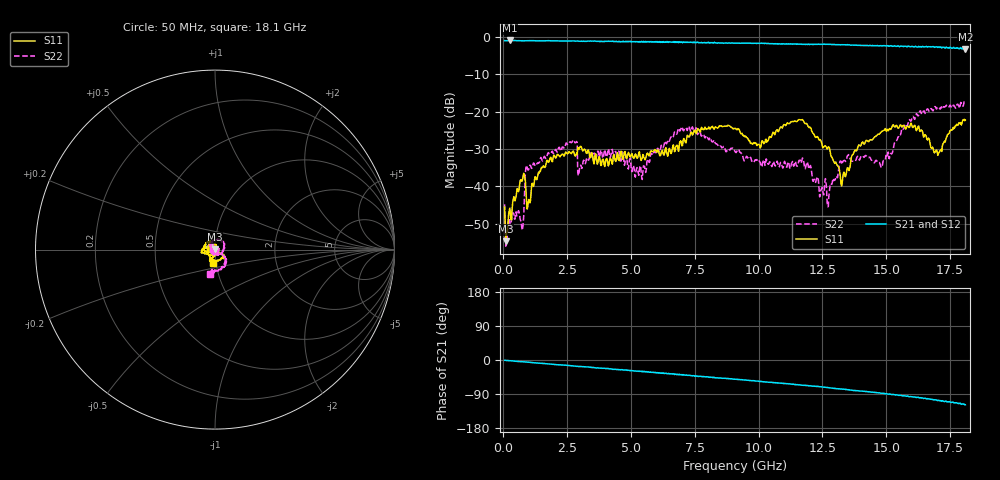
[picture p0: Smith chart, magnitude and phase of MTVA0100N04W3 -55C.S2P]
! Network Analyzer HP8720D.06.14 Serial No. US36140669
! 17 Jan 2005  10:34:37
! Frequency  S11  S21  S12  S22
# HZ  S  DB R 50
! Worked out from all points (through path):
!   801 points, 50 MHz to 18.1 GHz, reference 50 ohm
!   highest |S21| = -0.96 dB at 253.1 MHz (marker M1); lowest = -3.3 dB at 18.1 GHz (marker M2)
!   group delay of S21, straight-line fit = 17.1 ps
!   lowest |S11| = -54.7 dB at 95.12 MHz (marker M3), VSWR 1.00, Z = 49.8 + j0.0841 ohm
!   |S11| at or under -10 dB: start of sweep to end of sweep
!   |S22| runs from -56.0 to -17.0 dB; largest |S21 - S12| = 0.029
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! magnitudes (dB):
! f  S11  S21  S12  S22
! 50 MHz  -45.6  -1.0  -1.0  -44.8
! 95.12 MHz  -54.7  -1.0  -1.0  -56.0
! 253.1 MHz  -45.8  -1.0  -1.0  -49.7
! 726.9 MHz  -38.6  -1.1  -1.0  -51.2
! 975.1 MHz  -44.1  -1.0  -1.0  -35.6
! 1.765 GHz  -33.6  -1.0  -1.0  -31.0
! 2.69 GHz  -31.0  -1.1  -1.1  -28.2
! 3.073 GHz  -29.8  -1.2  -1.1  -35.2
! 4.179 GHz  -32.6  -1.2  -1.2  -32.3
! 5.375 GHz  -32.5  -1.4  -1.4  -34.5
! 6.074 GHz  -30.4  -1.4  -1.4  -30.1
! 7.202 GHz  -26.4  -1.4  -1.5  -25.1
! 9.075 GHz  -24.5  -1.7  -1.7  -30.6
! 10 GHz  -28.7  -1.7  -1.7  -33.0
! 12.1 GHz  -25.4  -2.0  -2.0  -37.4
! 12.75 GHz  -29.4  -2.0  -2.0  -42.5
! 13.29 GHz  -37.8  -2.1  -2.1  -33.4
! 13.99 GHz  -29.2  -2.3  -2.3  -32.2
! 15.1 GHz  -25.0  -2.5  -2.4  -32.4
! 16.05 GHz  -24.3  -2.6  -2.7  -21.3
! 16.97 GHz  -30.3  -2.7  -2.6  -19.3
! 18.1 GHz  -22.3  -3.3  -3.2  -17.0
